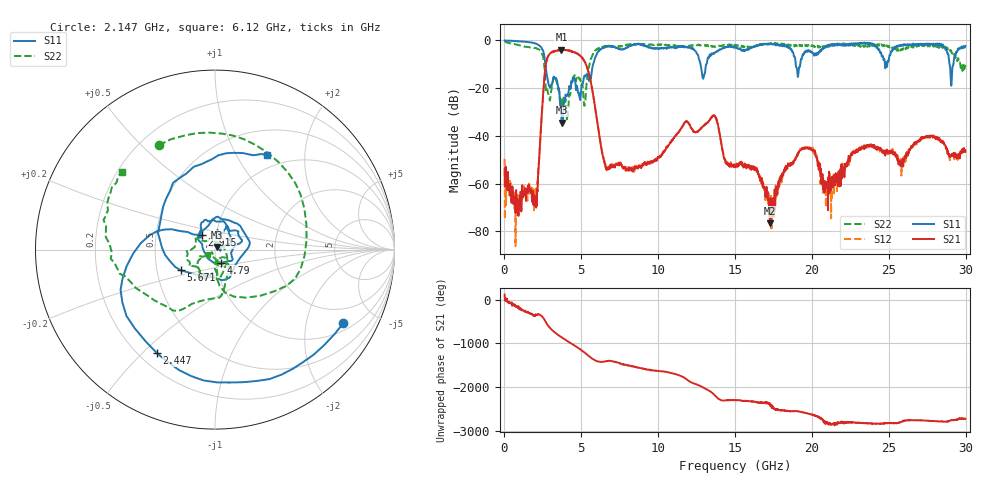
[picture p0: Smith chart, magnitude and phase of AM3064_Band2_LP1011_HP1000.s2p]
# Hz S DB R 50.0
!freq dBS11 angS11 dBS21 angS21 dBS12 angS12 dBS22 angS22
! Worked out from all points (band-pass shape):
!   1600 points, 10 MHz to 29.98 GHz, reference 50 ohm
!   highest |S21| = -3.86 dB at 3.703 GHz (marker M1); lowest = -76.5 dB at 17.29 GHz (marker M2)
!   |S21| within 3 dB of the highest: 2.825 GHz to 5.001 GHz (2.176 GHz wide, 55.6 % of centre)
!   lowest |S11| = -34.4 dB at 3.721 GHz (marker M3), VSWR 1.04, Z = 51.2 + j1.48 ohm
!   |S11| at or under -10 dB: 2.664 GHz to 5.77 GHz (3.106 GHz wide, 73.7 % of centre); 12.75 GHz to 13.13 GHz (378.6 MHz wide, 2.93 % of centre); 18.95 GHz to 19.24 GHz (294.4 MHz wide, 1.54 % of centre)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
!   |S22| runs from -33.1 to -0.3 dB; largest |S21 - S12| = 0.019
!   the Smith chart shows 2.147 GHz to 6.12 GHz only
!   S11 on the Smith chart (normalised r, x): 2.147 GHz: 1.29, -3.29; 2.447 GHz: 0.27, -0.56; 2.915 GHz: 0.85, +0.14; 4.79 GHz: 1.06, -0.15; 5.671 GHz: 0.66, -0.16; 6.12 GHz: 0.82, +1.35
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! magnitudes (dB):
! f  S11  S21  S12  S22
! 10 MHz  0.0  -53.6  -49.6  -0.3
! 797.2 MHz  -0.3  -71.0  -72.4  -1.8
! 2.147 GHz  -1.7  -63.4  -59.0  -3.6
! 2.447 GHz  -3.6  -29.0  -28.9  -5.8
! 2.915 GHz  -19.2  -5.8  -5.8  -24.0
! 3.703 GHz  -31.2  -3.9  -4.0  -24.7
! 3.721 GHz  -34.4  -4.1  -4.0  -25.2
! 4.79 GHz  -22.0  -5.8  -5.6  -15.7
! 5.015 GHz  -19.1  -7.1  -7.0  -18.9
! 5.671 GHz  -13.0  -19.4  -19.3  -7.1
! 6.12 GHz  -4.4  -37.7  -37.6  -3.4
! 6.72 GHz  -2.5  -53.9  -53.4  -2.3
! 10 GHz  -3.4  -48.8  -49.1  -1.9
! 13.6 GHz  -5.3  -31.7  -31.6  -2.5
! 15 GHz  -2.7  -53.0  -52.8  -1.9
! 17.29 GHz  -1.6  -76.5  -70.2  -1.3
! 19.99 GHz  -4.8  -45.6  -46.1  -2.0
! 20.89 GHz  -2.4  -61.7  -61.8  -2.8
! 25 GHz  -8.4  -46.7  -46.7  -2.3
! 28.28 GHz  -1.3  -41.7  -41.3  -3.1
! 29.08 GHz  -17.7  -48.5  -47.8  -5.2
! 29.98 GHz  -2.3  -46.7  -46.9  -10.2
